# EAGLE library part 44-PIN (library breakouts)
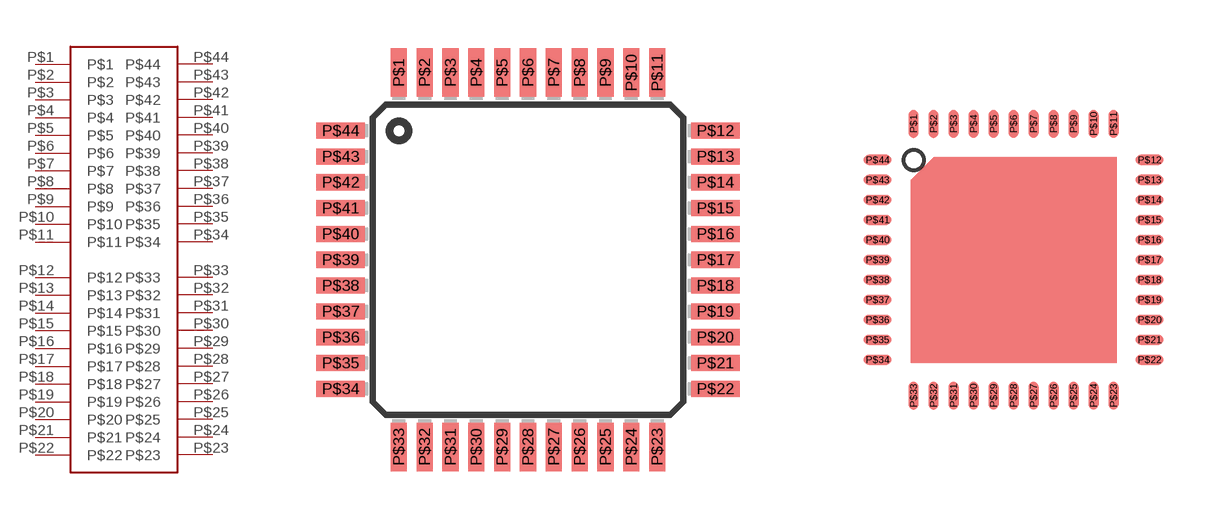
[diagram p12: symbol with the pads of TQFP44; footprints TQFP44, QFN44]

Designator prefix -

## 44-PINTQFP  [TQFP44]
P$1  P$1
P$2  P$2
P$3  P$3
P$4  P$4
P$5  P$5
P$6  P$6
P$7  P$7
P$8  P$8
P$9  P$9
P$10  P$10
P$11  P$11
P$12  P$12
P$13  P$13
P$14  P$14
P$15  P$15
P$16  P$16
P$17  P$17
P$18  P$18
P$19  P$19
P$20  P$20
P$21  P$21
P$22  P$22
P$23  P$23
P$24  P$24
P$25  P$25
P$26  P$26
P$27  P$27
P$28  P$28
P$29  P$29
P$30  P$30
P$31  P$31
P$32  P$32
P$33  P$33
P$34  P$34
P$35  P$35
P$36  P$36
P$37  P$37
P$38  P$38
P$39  P$39
P$40  P$40
P$41  P$41
P$42  P$42
P$43  P$43
P$44  P$44

## 44-PINQFN  [QFN44]
Pads as for TQFP44

## Footprint TQFP44 (pad centres in mm)
smd 0.5 x 1.5: P$1 -4,5.8; P$2 -3.2,5.8; P$3 -2.4,5.8; P$4 -1.6,5.8; P$5 -0.8,5.8; P$6 0,5.8; P$7 0.8,5.8; P$8 1.6,5.8; P$9 2.4,5.8; P$10 3.2,5.8; P$11 4,5.8; P$23 4,-5.8; P$24 3.2,-5.8; P$25 2.4,-5.8; P$26 1.6,-5.8; P$27 0.8,-5.8; P$28 0,-5.8; P$29 -0.8,-5.8; P$30 -1.6,-5.8; P$31 -2.4,-5.8; P$32 -3.2,-5.8; P$33 -4,-5.8
smd 1.5 x 0.5: P$12 5.8,4; P$13 5.8,3.2; P$14 5.8,2.4; P$15 5.8,1.6; P$16 5.8,0.8; P$17 5.8,0; P$18 5.8,-0.8; P$19 5.8,-1.6; P$20 5.8,-2.4; P$21 5.8,-3.2; P$22 5.8,-4; P$34 -5.8,-4; P$35 -5.8,-3.2; P$36 -5.8,-2.4; P$37 -5.8,-1.6; P$38 -5.8,-0.8; P$39 -5.8,0; P$40 -5.8,0.8; P$41 -5.8,1.6; P$42 -5.8,2.4; P$43 -5.8,3.2; P$44 -5.8,4

## Footprint QFN44 (pad centres in mm)
smd 0.25 x 0.7: P$1 -2.5,3.4; P$2 -2,3.4; P$3 -1.5,3.4; P$4 -1,3.4; P$5 -0.5,3.4; P$6 0,3.4; P$7 0.5,3.4; P$8 1,3.4; P$9 1.5,3.4; P$10 2,3.4; P$11 2.5,3.4; P$23 2.5,-3.4; P$24 2,-3.4; P$25 1.5,-3.4; P$26 1,-3.4; P$27 0.5,-3.4; P$28 0,-3.4; P$29 -0.5,-3.4; P$30 -1,-3.4; P$31 -1.5,-3.4; P$32 -2,-3.4; P$33 -2.5,-3.4
smd 0.7 x 0.25: P$12 3.4,2.5; P$13 3.4,2; P$14 3.4,1.5; P$15 3.4,1; P$16 3.4,0.5; P$17 3.4,0; P$18 3.4,-0.5; P$19 3.4,-1; P$20 3.4,-1.5; P$21 3.4,-2; P$22 3.4,-2.5; P$34 -3.4,-2.5; P$35 -3.4,-2; P$36 -3.4,-1.5; P$37 -3.4,-1; P$38 -3.4,-0.5; P$39 -3.4,0; P$40 -3.4,0.5; P$41 -3.4,1; P$42 -3.4,1.5; P$43 -3.4,2; P$44 -3.4,2.5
